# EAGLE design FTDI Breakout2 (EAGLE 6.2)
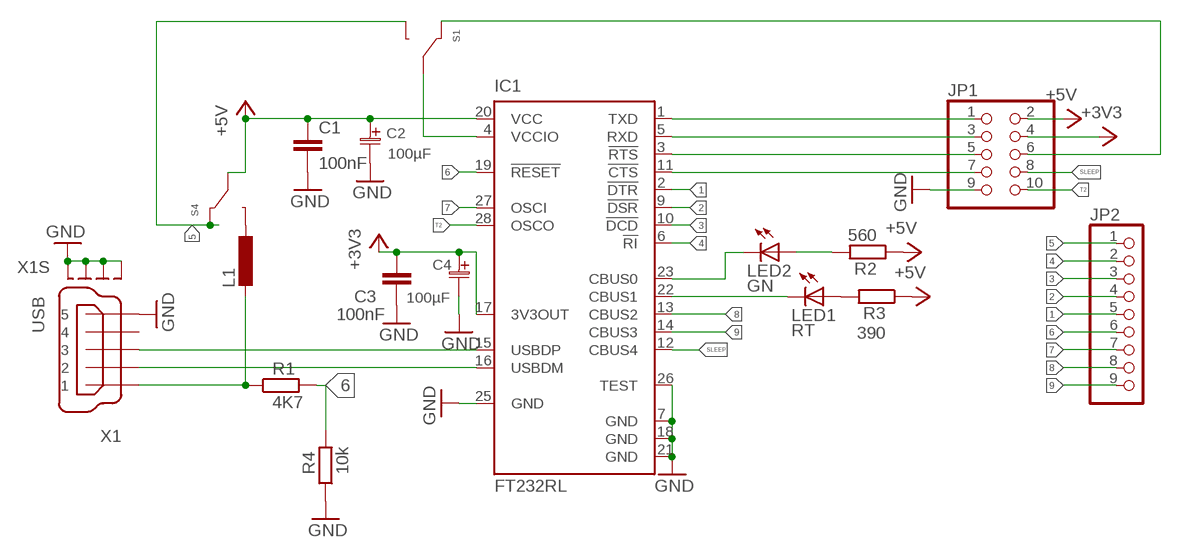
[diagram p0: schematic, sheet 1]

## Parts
C1  100nF  C-EUC0805  [C0805]
C2  100µF  ELKO_SMD-C  [SMD_C]
C3  100nF  C-EUC0805  [C0805]
C4  100µF  ELKO_SMD-C  [SMD_C]
IC1  FT232RL  [SSOP28]
JP1  PINHD-2X5  [2X05]
JP2  PINHD-1X9  [1X09]
L1  L-EUL2012C  [L2012C]
LED1  RT  LEDSML0603  [SML0603]
LED2  GN  LEDSML0603  [SML0603]
R1  4K7  R-EU_R0805  [R0805]
R2  560  R-EU_R0805  [R0805]
R3  390  R-EU_R0805  [R0805]
R4  10k  R-EU_R0805  [R0805]
S1  CAS120TB  [CAS120TB]
S4  CAS120TB  [CAS120TB]
X1  USB  MINI-USB_SHIELD5P4-32005-400  [32005-400]

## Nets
1: IC1.2(!DTR) JP2.5
2: IC1.9(!DSR) JP2.4
3: IC1.10(!DCD) JP2.3
4: IC1.6(!RI) JP2.2
5: JP2.1 S1.P$3 S4.P$1
6: IC1.19(!RESET) JP2.6 R1.2 R4.2
7: IC1.27(OSCI) JP2.7
8: IC1.13(CBUS2) JP2.8
9: IC1.14(CBUS3) JP2.9
+3V3: C3.1 C4.1(+) IC1.17(3V3OUT) JP1.4
+5V: C1.1 C2.1(+) IC1.20(VCC) JP1.2 R2.1 R3.1 S4.P$2
GND: C1.2 C2.2(-) C3.2 C4.2(-) IC1.7(GND) IC1.18(GND) IC1.21(GND) IC1.25(GND) IC1.26(TEST) JP1.9 R4.1 X1.5 X1.M1(S1) X1.M2(S2) X1.M3(S3) X1.M4(S4)
N$1: IC1.1(TXD) JP1.1
N$2: IC1.5(RXD) JP1.3
N$3: IC1.3(!RTS) JP1.5
N$4: IC1.11(!CTS) JP1.7
N$5: IC1.23(CBUS0) LED2.C
N$6: IC1.16(USBDM) X1.2
N$7: IC1.15(USBDP) X1.3
N$8: IC1.22(CBUS1) LED1.C
N$9: L1.2 R1.1 X1.1
N$10: L1.1 S4.P$3
N$11: LED1.A R3.2
N$12: LED2.A R2.2
N$17: IC1.4(VCCIO) S1.P$2
N$18: JP1.6 S1.P$1
SLEEP: IC1.12(CBUS4) JP1.8
T2: IC1.28(OSCO) JP1.10
Unconnected: X1.4

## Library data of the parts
C1 C3 = rcl:C-EU: CAPACITOR, European symbol
C2 C4 = Kapazitäten:ELKO
IC1 = ftdichip:FT232R: Source: http://www.ftdichip.com/Documents/DataSheets/DS_FT232R_v104.pdf; MPN: FT232RL; OC_FARNELL: 1146032; OC_NEWARK: 91K9918
JP1 = pinhead:PINHD-2X5: PIN HEADER
JP2 = pinhead:PINHD-1X9: PIN HEADER
L1 = rcl:L-EU: INDUCTOR, European symbol
LED1 LED2 = led:LED: LED
R1-R4 = rcl:R-EU_: RESISTOR, European symbol
S1 S4 = Selbst erstellt:CAS120TB
X1 = con-cypressindustries:MINI-USB_SHIELD5P4-: MINI USB-B R/A W/O POST 5 pol. Source: www.cypressindustries.com; OC_FARNELL: unknown; OC_NEWARK: unknown

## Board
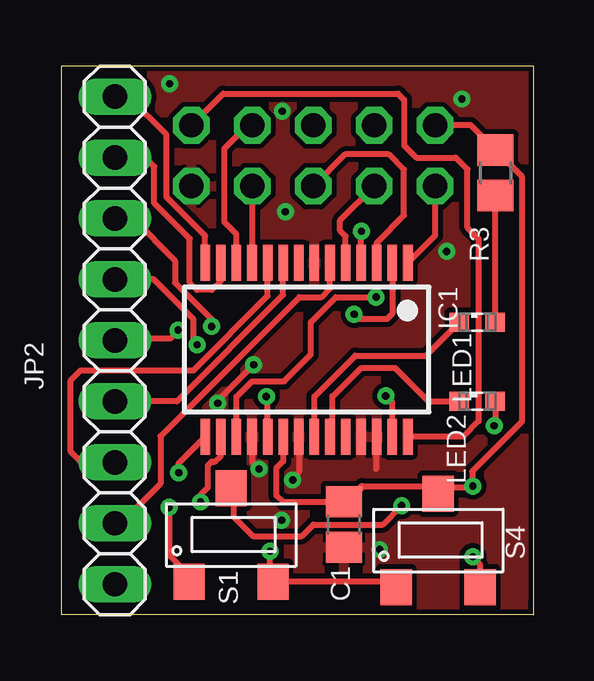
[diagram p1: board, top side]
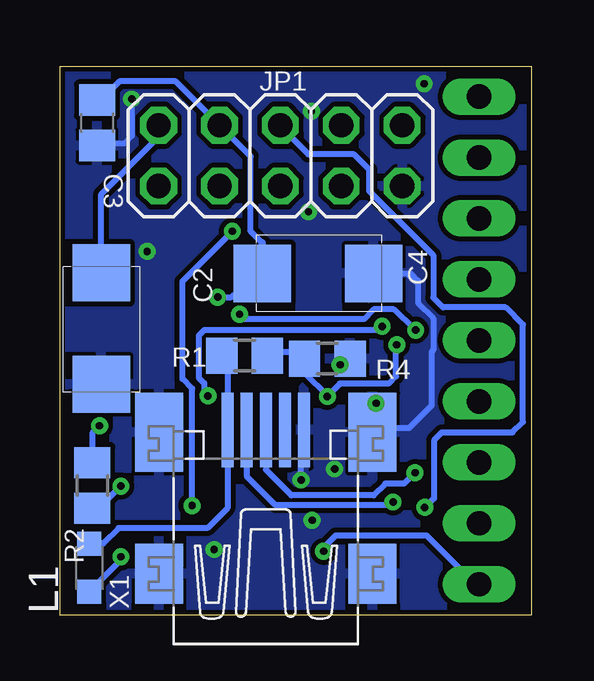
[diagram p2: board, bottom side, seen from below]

Size 19.68 x 22.89 mm. Coordinates in mm from the lower left corner, seen from the top.
Outline: 19.68,0.03 0,0.03 0,22.89 19.68,22.89 19.68,0
Copper layers (1*16): Top 0.035mm / dielectric 1.5mm / Bottom 0.035mm
Design rules: minimum track width 0.15mm, minimum drill 0.3mm, track to track 0.15mm, track to pad 0.15mm, pad to pad 0.15mm, via to via 0.15mm, smd to smd 0.15mm, copper to edge 0.15mm, drill to drill 0.2mm, minimum pad ring 0.15mm, minimum via ring 0.2mm, stop-mask expansion 0.15mm, vias tented up to drill 0.8mm, thermal gap 0.15mm

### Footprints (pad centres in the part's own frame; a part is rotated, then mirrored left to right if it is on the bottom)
C0805 = smd 1.3 x 1.5: 1 -0.95,0; 2 0.95,0
SMD_C = smd 2.388 x 2.388: 1 -2.311,0; 2 2.337,0
SSOP28 = smd 0.4 x 1.5: 1 -4.225,-3.625; 2 -3.575,-3.625; 3 -2.925,-3.625; 4 -2.275,-3.625; 5 -1.625,-3.625; 6 -0.975,-3.625; 7 -0.325,-3.625; 8 0.325,-3.625; 9 0.975,-3.625; 10 1.625,-3.625; 11 2.275,-3.625; 12 2.925,-3.625; 13 3.575,-3.625; 14 4.225,-3.625; 15 4.225,3.625; 16 3.575,3.625; 17 2.925,3.625; 18 2.275,3.625; 19 1.625,3.625; 20 0.975,3.625; 21 0.325,3.625; 22 -0.325,3.625; 23 -0.975,3.625; 24 -1.625,3.625; 25 -2.275,3.625; 26 -2.925,3.625; 27 -3.575,3.625; 28 -4.225,3.625
2X05 = drill 1.016 octagon: 1 -5.08,-1.27; 2 -5.08,1.27; 3 -2.54,-1.27; 4 -2.54,1.27; 5 0,-1.27; 6 0,1.27; 7 2.54,-1.27; 8 2.54,1.27; 9 5.08,-1.27; 10 5.08,1.27
1X09 = drill 1.016 long: 1 -10.16,0; 2 -7.62,0; 3 -5.08,0; 4 -2.54,0; 5 0,0; 6 2.54,0; 7 5.08,0; 8 7.62,0; 9 10.16,0
L2012C = smd 1 x 1: 1 -1,0; 2 1,0
SML0603 = smd 0.8 x 0.8: A 0.75,0; C -0.75,0
R0805 = smd 1.3 x 1.5: 1 -0.95,0; 2 0.95,0
CAS120TB = smd 1.3 x 1.5: P$1 -1.75,-1.95; P$2 0,1.95; P$3 1.75,-1.95
32005-400 = smd 3.1 x 0.5: 1 3,1.6; 2 3,0.8; 3 3,0; 4 3,-0.8; 5 3,-1.6 | smd 2.5 x 2: M1 -3,-4.45; M2 -3,4.45 | smd 3.3 x 2: M3 2.9,4.45; M4 2.9,-4.45

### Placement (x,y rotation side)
C1  11.76,3.78 270 top
C2  17.96,11.96 270 bottom
C3  18.14,20.52 270 bottom
C4  8.94,14.25 0 bottom
IC1  10.21,11.07 180 top
JP1  10.49,19.15 0 bottom
JP2  2.21,11.46 90 top
L1  18.47,1.98 90 bottom
LED1  17.32,12.22 0 top
LED2  17.32,8.92 0 top
R1  11.99,10.82 0 bottom
R2  18.34,5.41 90 bottom
R3  18.08,18.44 270 top
R4  8.53,10.69 180 bottom
S1  7.06,3.35 0 top
S4  15.7,3.12 0 top
X1  11.1,4.72 90 bottom

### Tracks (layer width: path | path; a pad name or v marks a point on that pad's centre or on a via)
1  (via drill 0.3)
  Top 0.254: IC1.2 13.79,12.57 13.56,12.34 12.39,12.34 v12.19,12.55 | v4.85,11.89 4.52,11.53 2.29,11.53 JP2.5
  Bottom 0.254: v4.85,11.89 4.93,11.94 5.77,12.75 6.6,12.75 7.01,12.34 11.99,12.34 v12.19,12.55
2
  Top 0.254: IC1.9 9.24,13.35 4.8,8.92 JP2.4
3
  Top 0.254: IC1.10 8.59,13.31 5.49,10.21 0.79,10.21 0.38,9.8 0.38,6.81 0.81,6.38 JP2.3
4
  Top 0.254: IC1.6 11.19,13.62 10.82,13.26 9.91,13.26 4.12,7.47 4.12,5.49 2.46,3.84 JP2.2
5  (via drill 0.3)
  Top 0.254: v8.69,2.67 8.69,1.53 S1.P$3 13.72,1.4 S4.P$1
  Bottom 0.254: v8.69,2.67 8.69,2.82 8.18,3.33 4.39,3.33 2.41,1.35 JP2.1
6  (via drill 0.3)
  Top 0.254: IC1.19 8.59,9.09 v8.53,9.12 | v5.64,11.28 5.49,11.43 5.49,12.34 3.81,14.02 2.23,14.02 JP2.6
  Bottom 0.254: v5.64,11.28 5.66,11.25 5.66,9.96 5.97,9.65 8.03,9.65 8.03,9.63 v8.53,9.12 8.53,9.14 9.48,10.09 R4.2 | 9.5,10.96 R4.2 | R1.2 11.19,10.97 9.76,10.97 R4.2
7  (via drill 0.3)
  Top 0.254: 13.72,7.52 IC1.27 13.79,8.87 v13.51,9.14 | v6.25,12.04 6.25,12.34 4.72,13.87 4.72,14.78 2.97,16.54 JP2.7
  Bottom 0.254: v6.25,12.04 6.25,11.89 13.66,11.89 13.89,11.66 13.89,9.91 13.66,9.68 13.66,9.3 v13.51,9.14
8
  Top 0.254: IC1.13 6.64,13.95 6.25,13.56 5.64,13.56 5.33,13.87 5.33,15.7 3.86,17.17 3.86,18.69 3.48,19.08 JP2.8
9
  Top 0.254: JP2.9 2.77,21.62 4.37,20.02 4.37,17.42 5.99,15.81 IC1.14
+3V3  (via drill 0.3)
  Top 0.254: IC1.17 7.29,9.11 7.92,9.75 9.27,9.75 10.39,10.87 10.39,12.22 11.43,13.26 v13.11,13.26
  Bottom 0.254: v13.11,13.26 12.55,13.26 C4.1 | 11.25,15.52 11.73,16 11.73,19.13 JP1.4 14.86,22.25 17.2,22.25 17.97,21.47 C3.1 17.59,21.47
  Bottom 0.305: C4.1 11.25,15.52
+5V  (via drill 0.3)
  Top 0.254: 11.96,4.8 11.9,4.73 C1.1 11.75,4.72 9.22,4.72 8.94,5 8.94,6.12 9.24,6.42 IC1.20 | JP1.2 17.05,20.42 R3.1 19.2,18.27 19.2,8.08 17.12,5.99 17.12,5.41 v17.14,5.39 17.09,5.33 15.96,5.33 S4.P$2 15.41,5.36 12.52,5.36
  Top 0.305: 12.52,5.36 11.96,4.8 11.73,4.57 | 11.47,5.03 C1.1
  Bottom 0.254: C2.1 17.96,17.55 15.57,19.94 JP1.2 | R2.1 18.09,4.44 v17.14,5.39
GND  (via drill 0.3)
  Top 0.254: IC1.26 13.11,7.42 13.11,6.1 | IC1.18 7.94,6.39 v8.23,6.1 | IC1.21 9.89,5.97 v9.63,5.64 | v6.5,8.84 6.5,8.97 6.53,8.97 v8,10.44
  Bottom 0.254: v9.63,5.64 9.63,7.6 X1.5 | 4.88,13.92 5.21,14.25 C4.2 5.05,14.25 4.75,13.94 4.75,13.01 4.12,12.37 4.12,11.05 4.19,10.97 4.19,8.74 5.13,7.8 6.48,7.8 X1.M4 6.65,8.69 v6.5,8.84 | R4.1 7.72,10.69 v8,10.44 | v16.69,21.51 16.69,19.96 16.99,19.66 18.05,19.66 C3.2
  other vias: 13.26,2.74 9.17,3.96 16.05,15.16 9.32,16.81 9.19,21.01 4.5,22.15
  pour Bottom (isolate 0.203): 0.1,0.1 0.05,23.01 19.66,22.94 19.61,0.1
  pour Top (isolate 0.203): -0.2,-0.13 -0.08,22.86 19.71,22.94 19.23,0.15
N$1
  Top 0.254: IC1.1 15.57,15.83 JP1.1
N$2
  Top 0.254: IC1.5 11.84,15.8 11.61,16.03 11.61,16.46 JP1.3
N$3
  Top 0.254: IC1.3 13.14,15.52 14.28,16.66 14.28,18.57 13.64,19.2 11.81,19.2 JP1.5
N$4
  Top 0.254: IC1.11 7.95,14.71 JP1.7
N$5
  Top 0.254: IC1.23 11.28,7.54 11.28,9.14 11.33,9.14 12.5,10.31 13.89,10.31 15.29,8.92 LED2.C
N$6  (via drill 0.3)
  Top 0.254: IC1.16 6.64,6.64 6.4,6.4 6.25,6.4 6.1,6.25 6.1,5.33 5.79,5.03 v5.79,4.72
  Bottom 0.254: X1.2 11.9,5.8 10.69,4.6 5.97,4.6 5.94,4.57 v5.79,4.72
N$7  (via drill 0.3)
  Top 0.254: v4.88,5.94 4.88,6.34 IC1.15
  Bottom 0.254: X1.3 11.1,6.07 10.03,5 6.6,5 6.12,5.49 5.33,5.49 v4.88,5.94
N$8
  Top 0.254: IC1.22 10.54,9.11 12.24,10.82 15.18,10.82 LED1.C
N$9
  Bottom 0.254: 18.46,2.97 L1.2 18.45,3 17.88,3 17.25,3.63 13.54,3.63 12.7,4.47 X1.1 12.7,10.58 R1.1
N$10  (via drill 0.3)
  Top 0.254: S4.P$3 17.45,2.11 v17.14,2.44
  Bottom 0.254: v17.14,2.44 17.14,2.3 L1.1
N$11
  Top 0.254: LED1.A 18.07,17.5 | 17.98,17.68 18.07,17.59 18.07,17.5 | 18.07,17.5 R3.2
N$12  (via drill 0.3)
  Top 0.254: LED2.A 18.07,7.94 v18.03,7.9
  Bottom 0.254: R2.2 18.31,7.62 v18.03,7.9
N$17  (via drill 0.3)
  Top 0.254: IC1.4 12.49,15.99 v12.5,16 | v14.17,4.57 13.39,3.78 10.49,3.78 10.01,3.3 7.98,3.3 7.16,4.12 7.16,5.2 S1.P$2
  Bottom 0.254: v12.5,16 14.58,13.92 14.58,9.86 14.17,9.45 v14.17,4.57
N$18  (via drill 0.3)
  Top 0.254: v4.47,4.5 4.47,2.51 5.31,1.67 S1.P$1 5.33,1.42 5.33,1.37 5.49,1.22 5.46,1.22
  Bottom 0.254: JP1.6 10.49,20.37 9.32,19.2 7.42,19.2 6.78,18.57 6.78,17.68 4.12,15.01 4.12,13.23 3.71,12.83 1.09,12.83 0.38,12.12 0.38,8.05 0.81,7.62 3.76,7.62 4.09,7.29 4.09,4.88 v4.47,4.5
SLEEP
  Top 0.254: IC1.12 7.29,15.88 6.78,16.38 6.78,19.46 7.75,20.42 JP1.8
T2
  Top 0.254: IC1.28 16.75,7.45 17.37,8.08 17.37,15.7 16.92,16.15 16.92,18.59 16.43,19.08 14.78,19.08 14.28,19.58 14.28,21.49 14.02,21.74 6.73,21.74 JP1.10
